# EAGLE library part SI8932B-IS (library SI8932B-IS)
Isolation Amplifiers Isolated voltage sensor with single ended input and single ended output. Narrow body S08. Source: Datasheet
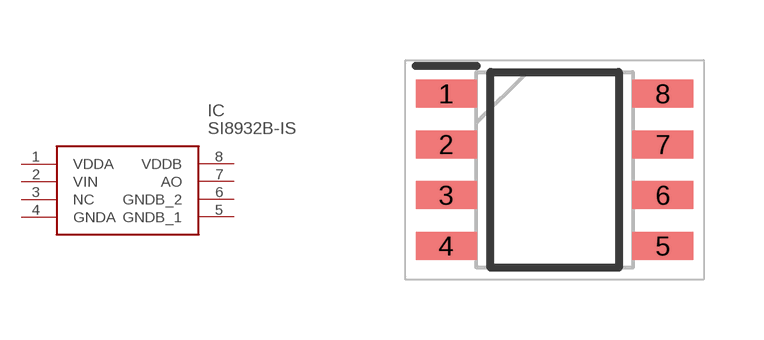
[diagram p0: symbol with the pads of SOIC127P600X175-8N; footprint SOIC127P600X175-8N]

Designator prefix IC

## SI8932B-IS (Description: Isolation Amplifiers Isolated voltage sensor with single ended input and single ended output. Narrow body S08.; Height: 1.75mm; Manufacturer_Name: Skyworks; Manufacturer_Part_Number: SI8932B-IS; Mouser_Part_Number: 873-SI8932B-IS; Mouser_Price-Stock: https://www.mouser.co.uk/ProductDetail/Skyworks-Solutions-Inc/SI8932B-IS?qs=yqaQSyyJnNgaRLq9HA2Jow%3D%3D)  [SOIC127P600X175-8N]
1  VDDA
2  VIN
3  NC  nc
4  GNDA
5  GNDB_1
6  GNDB_2
7  AO
8  VDDB

## Footprint SOIC127P600X175-8N (pad centres in mm)
8-Pin Narrow Body SOIC
smd 1.525 x 0.7: 1 -2.712,1.905; 2 -2.712,0.635; 3 -2.712,-0.635; 4 -2.712,-1.905; 5 2.712,-1.905; 6 2.712,-0.635; 7 2.712,0.635; 8 2.712,1.905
